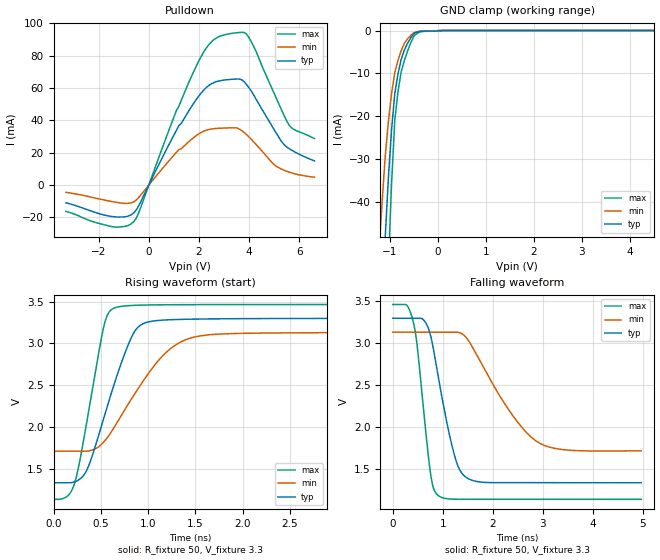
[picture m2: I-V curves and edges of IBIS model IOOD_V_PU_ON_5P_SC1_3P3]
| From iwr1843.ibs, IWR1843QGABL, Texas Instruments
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|   Model Cell IOOD_V_PU_ON_5P_SC1_3P3
|IOOD_V_PU_ON_5P_SC1_3P3
[Model]   IOOD_V_PU_ON_5P_SC1_3P3
Model_type   I/O_open_drain
Polarity   Non-Inverting
Enable   Active-Low
Vinl =  0.8V
Vinh =  2V
Cref =  15pF
Rref =  100.0000M
Vref =  0V
Vmeas =  1.65
|   typ   min   max
C_comp   2.059994p   1.862014p   2.067327p
[Model Spec]
Vinl   0.8V   0.8V   0.8V
Vinh   2V   2V   2V
[Temperature Range]   25   125   -40
[Voltage Range]   3.3   3.135   3.465
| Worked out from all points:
|   slope of the pulldown table from 0 to 0.495 V, typ, clamps not added: 31.8 ohm
|   GND clamp passes 1 mA (typ) near -0.52 V on its own axis
|   rising waveform, R_fixture 50, V_fixture 3.3: 20-80 % time 333ps typ, 511ps min, 217ps max; typ from 1.34 V to 3.3 V
|   falling waveform, R_fixture 50, V_fixture 3.3: 20-80 % time 385ps typ, 889ps min, 239ps max; typ from 3.3 V to 1.34 V
| Where Nom  PVT is Nominal Process, 3.3V, 25C
|   Fast PVT is Strong Process,  3.465V, -40C
|   Slow PVT is Weak Process,   3.135V, 125C
[Pulldown]
|   voltage   I(typ)   I(min)   I(max)
-3.3V     -10.93mA   -4.474mA   -16.27mA
-1.4V     -19.53mA   -10.38mA   -25.83mA
-600mV    -17.23mA   -10.34mA   -22.61mA
1.2V      36.72mA    21.93mA    48.77mA
1.9V      53.02mA    30.66mA    73.76mA
2.4V      61.61mA    34.34mA    86.89mA
3V        64.86mA    35.24mA    92.76mA
3.6V      65.51mA    34.65mA    94.24mA
3.9V      62.01mA    31.1mA     93.16mA
5V        34.1mA     12.57mA    56.41mA
5.6V      22.42mA    7.958mA    36.79mA
6.6V      14.97mA    4.886mA    28.74mA
[GND_clamp]
|   voltage   I(typ)   I(min)   I(max)
-3.3V     -787.2mA   -627.7mA   -1.235A
-1.233V   -85.67mA   -52.14mA   -138.8mA
-1.167V   -66.48mA   -40.37mA   -107.8mA
-1.1V     -48.26mA   -29.38mA   -78.01mA
-1.033V   -34.3mA    -21.2mA    -54.61mA
-966.7mV  -23.1mA    -14.68mA   -35.59mA
-900mV    -14.66mA   -9.807mA   -20.94mA
-833.3mV  -10.12mA   -6.96mA    -14.29mA
-700mV    -4.501mA   -2.971mA   -6.963mA
-500mV    -717.7uA   -493.4uA   -1.262mA
100mV     0A         0A         0A
6.6V      0A         0A         0A
[Ramp]
| variable   typ   min   max
dV/dt_f  1.1795006/0.38538225n 0.85573709/0.89559792n  1.3970808/0.23966865n
dV/dt_r  1.1738038/0.46664243n 0.86214199/1.0172278n  1.4060326/0.25228723n
R_load = 50
[Rising Waveform]
R_fixture = 50
V_fixture = 3.3
V_fixture_min = 3.135
V_fixture_max = 3.465
|   time   V(typ)   V(min)   V(max)
0s        1.338V     1.715V     1.141V
139.3ps   1.338V     1.715V     1.172V
221.2ps   1.349V     1.715V     1.327V
355ps     1.496V     1.716V     2.084V
528.3ps   2.097V     1.821V     3.184V
640.2ps   2.509V     1.996V     3.422V
905.9ps   3.206V     2.481V     3.457V
1.197ns   3.282V     2.899V     3.462V
1.482ns   3.29V      3.074V     3.463V
4.974ns   3.3V       3.133V     3.465V
[Falling Waveform]
R_fixture = 50
V_fixture = 3.3
V_fixture_min = 3.135
V_fixture_max = 3.465
|   time   V(typ)   V(min)   V(max)
0s        3.3V       3.134V     3.464V
277.3ps   3.3V       3.134V     3.457V
413.4ps   3.3V       3.134V     3.247V
752.8ps   3.102V     3.134V     1.456V
904.2ps   2.62V      3.134V     1.188V
1.248ns   1.635V     3.134V     1.142V
1.515ns   1.385V     3.033V     1.141V
2.314ns   1.339V     2.213V     1.14V
2.895ns   1.339V     1.825V     1.14V
4.974ns   1.338V     1.718V     1.14V
